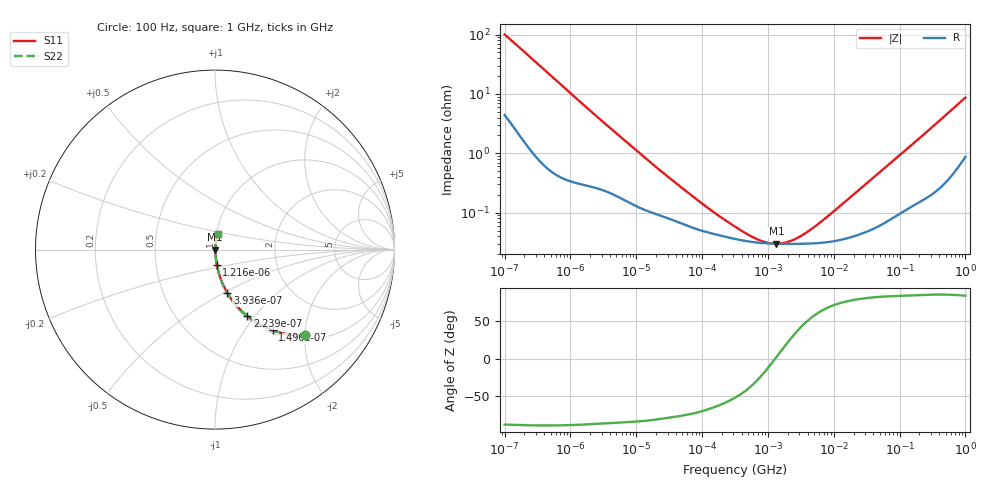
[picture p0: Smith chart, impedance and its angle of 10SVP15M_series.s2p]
!  *** S-Parameter ***
!  Copyright (C) Panasonic Industry Corporation
!  Conductive Polymer Aluminum Soild Capacitor (OS-CON)
!  Parts No. 10SVP15M
!  Connection Mode : Series
!  1  o---||---o  2
!  GND o--------o GND
!  Conditions : Temperature = 20 degC  DC Bias = 0 V
! Frequency Range : 100Hz  -  1GHz  [ 401 Steps ]
# Hz S RI R 50
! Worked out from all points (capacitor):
!   401 points, 100 Hz to 1 GHz, reference 50 ohm
!   read as one part in series: C = 15.7 uF near 108.4 Hz
!   lowest |Z| = 30 mohm at 1.349 MHz (marker M1)
!   series resonance near 1.28 MHz, so ESL is about 980 pH
!   S11 on the Smith chart (normalised r, x): 100 Hz: 1.09, -2.01; 149.6 Hz: 1.05, -1.36; 223.9 Hz: 1.03, -0.91; 393.6 Hz: 1.01, -0.52; 1.216 kHz: 1.01, -0.17; 1 GHz: 1.02, +0.17
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100  0.5026 -0.4785  0.4974 0.4785  0.4974 0.4785  0.5026 -0.4785
149.6236  0.3216 -0.4497  0.6784 0.4497  0.6784 0.4497  0.3216 -0.4497
223.8721  0.1794 -0.3697  0.8206 0.3697  0.8206 0.3697  0.1794 -0.3697
393.5501  0.0687 -0.2412  0.9313 0.2412  0.9313 0.2412  0.0687 -0.2412
664.5077  0.0272 -0.1499  0.9728 0.1499  0.9728 0.1499  0.0272 -0.1499
1216.186  0.0102 -0.0838  0.9898 0.0838  0.9898 0.0838  0.0102 -0.0838
1487.647  0.00775 -0.0689  0.9922 0.0689  0.9922 0.0689  0.00775 -0.0689
4241.31  0.00271 -0.0251  0.9973 0.0251  0.9973 0.0251  0.00271 -0.0251
22130.95  0.000936 -0.00526  0.9991 0.00526  0.9991 0.00526  0.000936 -0.00526
110917.5  0.00048 -0.00121  0.9995 0.00121  0.9995 0.00121  0.00048 -0.00121
316227.8  0.000361 -0.000456  0.9996 0.000456  0.9996 0.000456  0.000361 -0.000456
737055.2  0.000311 -0.000149  0.9997 0.000149  0.9997 0.000149  0.000311 -0.000149
1017419  0.000303 -6.02e-05  0.9997 6.02e-05  0.9997 6.02e-05  0.000303 -6.02e-05
1348963  0.0003 1.38e-05  0.9997 -1.38e-05  0.9997 -1.38e-05  0.0003 1.38e-05
1788546  0.000298 8.95e-05  0.9997 -8.95e-05  0.9997 -8.95e-05  0.000298 8.95e-05
2371374  0.000297 0.000173  0.9997 -0.000173  0.9997 -0.000173  0.000297 0.000173
3273407  0.000299 0.000285  0.9997 -0.000285  0.9997 -0.000285  0.000299 0.000285
4704354  0.000303 0.000447  0.9997 -0.000447  0.9997 -0.000447  0.000303 0.000447
9716280  0.000329 0.000971  0.9997 -0.000971  0.9997 -0.000971  0.000329 0.000971
6.99842e7  0.000791 0.00657  0.9992 -0.00657  0.9992 -0.00657  0.000791 0.00657
3.368992e8  0.00304 0.0295  0.997 -0.0295  0.997 -0.0295  0.00304 0.0295
1e9  0.0159 0.0845  0.9841 -0.0845  0.9841 -0.0845  0.0159 0.0845
